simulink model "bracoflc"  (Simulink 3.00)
settings: Solver=ode45  StartTime=0.0  StopTime=15  MaxStep=0.005  RelTol=1e-3  AbsTol=1e-3

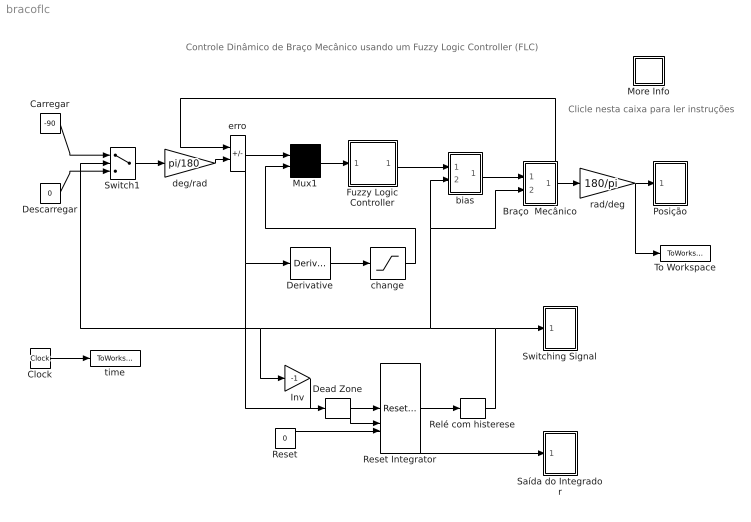
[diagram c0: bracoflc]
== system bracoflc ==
  note: Controle Dinâmico de Braço Mecânico usando um Fuzzy Logic Controller (FLC)
  note: Clicle nesta caixa para ler instruções
  Braço  Mecânico : Subsystem
      mask help: Braço mecânico
      mask init:
      | m1=@1;ml=@2;a1=@3;b1=@4;g=@5;xi=@6;
  Carregar : Constant  Value=-90
  Clock : Clock
  Dead Zone : DeadZone  LowerValue=-3/180*pi  UpperValue=3/180*pi
  Derivative : Derivative
  Descarregar : Constant  Value=0
  Fuzzy Logic Controller : Subsystem  mask(FIS){}
      mask help: FIS
      mask init:
      | fismatrix = @1;
  Inv : Gain  Gain=-1  SaturateOnIntegerOverflow=on
  More Info : Subsystem
  Mux1 : Mux  Inputs=2
  Posição : Subsystem  mask(Storage scope.){}
      mask help: Storage scope using MATLAB graph window. Enter plotting ranges and line type.
      mask init:
      | npts = @4; color = @5; ax = [0, @1, @2, @3]; dt=-1;
  Relé com histerese : Relay  OnSwitchValue=1  OffSwitchValue=-1  OnOutputValue=1  OffOutputValue=-1
  Reset : Constant  Value=0
  Reset Integrator : ResetIntegrator  InitialCondition=1
  Saída do Integrador : Subsystem  mask(Storage scope.){}
      mask help: Storage scope using MATLAB graph window. Enter plotting ranges and line type.
      mask init:
      | npts = @4; color = @5; ax = [0, @1, @2, @3]; dt=-1;
  Switch1 : Switch  Threshold=0
  Switching Signal : Subsystem  mask(Storage scope.){}
      mask help: Storage scope using MATLAB graph window. Enter plotting ranges and line type.
      mask init:
      | npts = @4; color = @5; ax = [0, @1, @2, @3]; dt=-1;
  To Workspace : ToWorkspace  VariableName=teta  SampleTime=0  SaveFormat=Matrix
  bias : Subsystem
      mask help: Bias
      mask init:
      | m1=@1;ml=@2;a1=@3;g=@4;
  change : Saturate  UpperLimit=10  LowerLimit=-10
  deg/rad : Gain  Gain=pi/180  SaturateOnIntegerOverflow=on
  erro : Sum  Inputs=-+  SaturateOnIntegerOverflow=on
  rad/deg : Gain  Gain=180/pi  SaturateOnIntegerOverflow=on
  time : ToWorkspace  VariableName=t  SampleTime=0  SaveFormat=Matrix
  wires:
  Reset/1 -> Reset Integrator/3
  Dead Zone/1 -> Reset Integrator/2
  Clock/1 -> time/1
  Switch1/1 -> deg/rad/1
  rad/deg/1 -> Posição/1(x), To Workspace/1
  deg/rad/1 -> erro/2
  Braço  Mecânico/1(ângulo do braço) -> rad/deg/1, erro/1
  Inv/1 -> Reset Integrator/1
  bias/1(biased control) -> Braço  Mecânico/1(torque)
  Descarregar/1 -> Switch1/3
  Carregar/1 -> Switch1/1
  Reset Integrator/1 -> Relé com histerese/1, Saída do Integrador/1(x)
  Derivative/1 -> change/1
  Mux1/1 -> Fuzzy Logic Controller/1(In1)
  Fuzzy Logic Controller/1(Out1) -> bias/1(unbiased control)
  erro/1 -> Mux1/1, Dead Zone/1, Derivative/1
  change/1 -> Mux1/2
  Relé com histerese/1 -> Switching Signal/1(x), Switch1/2, Inv/1, bias/2("toggle "), Braço  Mecânico/2(carga/descarga)

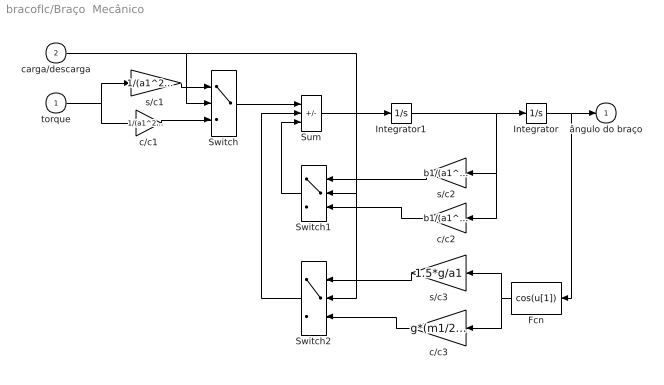
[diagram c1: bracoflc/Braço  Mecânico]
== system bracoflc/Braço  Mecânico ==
  torque : Inport  Port=1  PortWidth=-1  SampleTime=-1  DataType=auto
  carga/descarga : Inport  Port=2  PortWidth=-1  SampleTime=-1  DataType=auto
  Fcn : Fcn  Orientation=left  Expr=cos(u[1])
  Integrator : Integrator  ExternalReset=none  InitialConditionSource=internal  InitialCondition=xi(1)  LimitOutput=off  UpperSaturationLimit=inf  LowerSaturationLimit=-inf  ShowSaturationPort=off  ShowStatePort=off  AbsoluteTolerance=auto
  Integrator1 : Integrator  ExternalReset=none  InitialConditionSource=internal  InitialCondition=xi(2)  LimitOutput=off  UpperSaturationLimit=inf  LowerSaturationLimit=-inf  ShowSaturationPort=off  ShowStatePort=off  AbsoluteTolerance=auto
  Sum : Sum  Inputs=+--  SaturateOnIntegerOverflow=on
  Switch : Switch  Threshold=0
  Switch1 : Switch  Orientation=left  Threshold=0
  Switch2 : Switch  Orientation=left  Threshold=0
  c/c1 : Gain  Gain=1/(a1^2*(m1/3+ml))  SaturateOnIntegerOverflow=on
  c/c2 : Gain  Orientation=left  Gain=b1/(a1^2*(m1/3+ml))  SaturateOnIntegerOverflow=on
  c/c3 : Gain  Orientation=left  Gain=g*(m1/2+ml)/(a1*(m1/3+ml))  SaturateOnIntegerOverflow=on
  "s/c1 " : Gain  Gain=1/(a1^2*m1/3)  SaturateOnIntegerOverflow=on
  s/c2 : Gain  Orientation=left  Gain=b1/(a1^2*m1/3)  SaturateOnIntegerOverflow=on
  s/c3 : Gain  Orientation=left  Gain=1.5*g/a1  SaturateOnIntegerOverflow=on
  ângulo do braço : Outport  Port=1
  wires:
  Switch/1 -> Sum/1
  carga/descarga/1 -> Switch/2, Switch2/2, Switch1/2
  torque/1 -> "s/c1 "/1, c/c1/1
  Switch1/1 -> Sum/3
  c/c1/1 -> Switch/3
  s/c3/1 -> Switch2/1
  s/c2/1 -> Switch1/1
  "s/c1 "/1 -> Switch/1
  Sum/1 -> Integrator1/1
  Integrator/1 -> ângulo do braço/1, Fcn/1
  Integrator1/1 -> Integrator/1, c/c2/1, s/c2/1
  c/c3/1 -> Switch2/3
  Switch2/1 -> Sum/2
  c/c2/1 -> Switch1/3
  Fcn/1 -> s/c3/1, c/c3/1

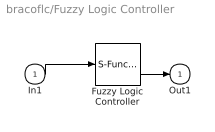
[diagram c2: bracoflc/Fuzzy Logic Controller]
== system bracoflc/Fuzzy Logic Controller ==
  In1 : Inport  Port=1  PortWidth=-1  SampleTime=-1  DataType=auto
  Fuzzy Logic Controller : S-Function  FunctionName=sffis  Parameters=fismatrix  PortCounts=[]  SFunctionModules=''
  Out1 : Outport  Port=1
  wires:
  In1/1 -> Fuzzy Logic Controller/1
  Fuzzy Logic Controller/1 -> Out1/1

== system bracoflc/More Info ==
  note: Para executar esta simulação: 1) certifique-se que o arquivo "bracoflc.fis" está no seu diretório atual; 2) no prompt do MATLAB execute: BRACO=readfis('bracoflc'); 3) rode esta simulação escolhendo no menu as opções: Simulation/Start; 4) ajuste os valores em Simulation/Parameters se necessário. Cairo L. Nascimento Jr. - ITA - cairo@ita.br Agradecimentos são devidos a Tibério Augusto de Melo e Roberto Kawakami Harrop Galvão

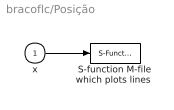
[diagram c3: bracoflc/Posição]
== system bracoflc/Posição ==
  x : Inport  Port=1  PortWidth=-1  SampleTime=-1  DataType=auto
  "S-function M-file which plots lines " : S-Function  FunctionName=sfunyst  Parameters=ax, color, npts, dt  PortCounts=[]  SFunctionModules=''
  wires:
  x/1 -> "S-function M-file which plots lines "/1

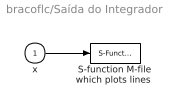
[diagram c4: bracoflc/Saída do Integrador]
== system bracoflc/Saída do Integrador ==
  x : Inport  Port=1  PortWidth=-1  SampleTime=-1  DataType=auto
  "S-function M-file which plots lines " : S-Function  FunctionName=sfunyst  Parameters=ax, color, npts, dt  PortCounts=[]  SFunctionModules=''
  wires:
  x/1 -> "S-function M-file which plots lines "/1

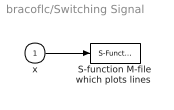
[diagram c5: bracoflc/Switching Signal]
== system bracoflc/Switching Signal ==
  x : Inport  Port=1  PortWidth=-1  SampleTime=-1  DataType=auto
  "S-function M-file which plots lines " : S-Function  FunctionName=sfunyst  Parameters=ax, color, npts, dt  PortCounts=[]  SFunctionModules=''
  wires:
  x/1 -> "S-function M-file which plots lines "/1

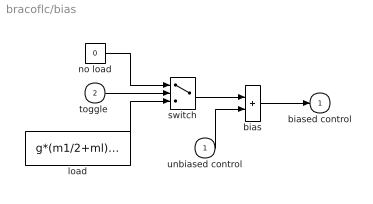
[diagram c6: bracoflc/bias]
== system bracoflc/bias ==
  unbiased control : Inport  Port=1  PortWidth=-1  SampleTime=-1  DataType=auto
  "toggle " : Inport  Port=2  PortWidth=-1  SampleTime=-1  DataType=auto
  bias : Sum  Inputs=++  SaturateOnIntegerOverflow=on
  load : Constant  Value=g*(m1/2+ml)*a1
  no load : Constant  Value=0
  switch : Switch  Threshold=0
  biased control : Outport  Port=1
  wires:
  unbiased control/1 -> bias/2
  "toggle "/1 -> switch/2
  bias/1 -> biased control/1
  switch/1 -> bias/1
  no load/1 -> switch/1
  load/1 -> switch/3
